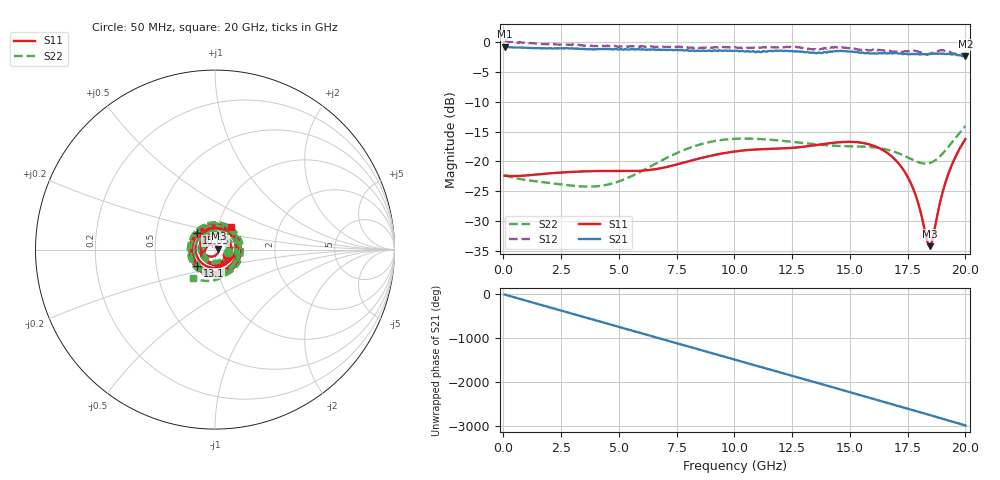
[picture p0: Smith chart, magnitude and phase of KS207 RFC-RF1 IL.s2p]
!Agilent	"Technologies,E8364B,MY43040668,A.07.50.67"
!Agilent	E8364B:	A.07.50.67
!Date:	"Friday,"	June	"03,"	2022	13:34:58
!Correction:	S11(Full	2	"Port(1,2))"
!S21(Full	2	"Port(1,2))"
!S12(Full	2	"Port(1,2))"
!S22(Full	2	"Port(1,2))"
!S2P	File:	Measurements:	"S11,"	"S21,"	"S12,"	S22:
#	Hz	S	dB	R	50
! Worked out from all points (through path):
!   400 points, 50 MHz to 20 GHz, reference 50 ohm
!   highest |S21| = -0.76 dB at 50 MHz (marker M1); lowest = -2.4 dB at 20 GHz (marker M2)
!   group delay of S21, straight-line fit = 414 ps
!   lowest |S11| = -34.2 dB at 18.45 GHz (marker M3), VSWR 1.04, Z = 51.9 + j0.49 ohm
!   |S11| at or under -10 dB: start of sweep to end of sweep
!   |S22| runs from -24.2 to -14.1 dB; largest |S21 - S12| = 0.12
!   S11 on the Smith chart (normalised r, x): 50 MHz: 1.15, -0.07; 13.1 GHz: 0.81, -0.15; 15.85 GHz: 0.80, +0.15; 20 GHz: 1.15, +0.30
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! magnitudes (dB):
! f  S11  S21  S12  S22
! 50 MHz  -22.4  -0.8  0.3  -22.3
! 1 GHz  -22.3  -0.9  -0.1  -23.1
! 3.4 GHz  -21.7  -1.1  -0.5  -24.2
! 4.85 GHz  -21.6  -1.1  -0.6  -23.5
! 6.7 GHz  -21.2  -1.2  -0.8  -20.1
! 8.45 GHz  -19.5  -1.4  -1.0  -17.2
! 10.05 GHz  -18.3  -1.4  -0.9  -16.2
! 13.1 GHz  -17.5  -1.7  -1.0  -17.0
! 13.35 GHz  -17.4  -1.7  -1.2  -17.1
! 14.85 GHz  -16.7  -1.5  -0.9  -17.4
! 15.85 GHz  -17.1  -1.9  -1.4  -17.6
! 16.7 GHz  -18.8  -1.8  -1.5  -18.1
! 17.2 GHz  -20.8  -1.9  -1.6  -18.8
! 17.65 GHz  -23.7  -2.0  -1.4  -19.6
! 17.95 GHz  -26.9  -2.0  -1.6  -20.1
! 18.35 GHz  -33.4  -2.0  -2.1  -20.3
! 18.45 GHz  -34.2  -1.9  -2.0  -20.3
! 18.55 GHz  -33.5  -1.9  -1.8  -20.1
! 18.9 GHz  -26.9  -1.9  -1.4  -19.1
! 19.2 GHz  -22.8  -2.0  -1.5  -17.8
! 19.55 GHz  -19.4  -2.0  -1.9  -16.2
! 20 GHz  -16.3  -2.4  -1.9  -14.1
